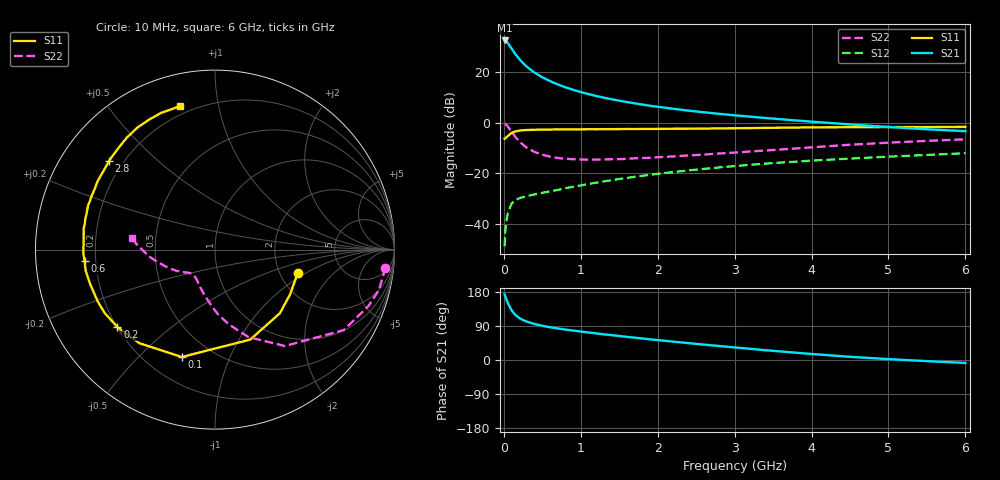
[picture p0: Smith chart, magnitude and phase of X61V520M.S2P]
! SIEMENS Small Signal Semiconductors
! BFP193W
! Si NPN RF Bipolar Junction Transistor in SOT343
! VCE = 1.5 V  IC = 20 mA
! Common Emitter S-Parameters:  April 1994
# GHz  S  MA  R  50
!  f  S11  S21  S12  S22
! GHz  MAG  ANG  MAG  ANG  MAG  ANG  MAG  ANG
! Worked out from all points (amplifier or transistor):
!   40 points, 10 MHz to 6 GHz, reference 50 ohm
!   highest |S21| = 32.5 dB at 10 MHz (marker M1)
!   |S21| within 3 dB of that: start of sweep to 96.08 MHz
!   unconditionally stable (mu >= 1): 873.5 MHz to 4.167 GHz
!   at 200 MHz: K = 0.36, MSG = 27.6 dB, |S12| = -30.0 dB
!   at 1.5 GHz: K = 1.13, MAG = 13.3 dB, |S12| = -22.3 dB
!   at 6 GHz: K = 0.95, MSG = 4.4 dB, |S12| = -12.1 dB
!   S11 on the Smith chart (normalised r, x): 10 MHz: 2.52, -0.84; 100 MHz: 0.34, -0.68; 200 MHz: 0.20, -0.34; 600 MHz: 0.16, -0.04; 2.8 GHz: 0.15, +0.36; 6 GHz: 0.16, +0.78
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0.01  0.4794 -15.5  42.23 173.0  0.0036 83.6  0.9545 -6.0
0.02  0.4869 -30.7  41.82 167.6  0.0073 77.8  0.9412 -13.7
0.03  0.5064 -44.4  40.79 161.7  0.0105 75.2  0.9115 -20.1
0.05  0.5384 -68.6  37.76 150.9  0.016 64.5  0.8462 -32.0
0.1  0.6264 -107.2  29.31 131.2  0.0249 50.1  0.6631 -54.1
0.15  0.671 -129.1  22.71 118.7  0.0294 42.0  0.5215 -69.1
0.2  0.6942 -141.6  18.13 110.8  0.0318 38.7  0.4261 -79.2
0.25  0.7091 -150.1  15.05 105.3  0.0338 37.4  0.3644 -86.9
0.3  0.7145 -156.2  12.72 101.2  0.0353 36.8  0.317 -93.1
0.4  0.722 -164.9  9.753 94.9  0.038 37.8  0.2627 -102.5
0.5  0.7298 -170.5  7.897 90.3  0.0408 40.1  0.2317 -109.6
0.6  0.7298 -175.0  6.608 86.5  0.0438 42.1  0.212 -115.3
0.8  0.7328 178.4  5 80.3  0.0504 46.4  0.1927 -123.0
1.1  0.7411 170.9  3.676 72.6  0.0612 50.2  0.185 -130.5
1.3  0.7427 166.5  3.118 67.7  0.0688 51.9  0.187 -133.6
1.6  0.7489 160.5  2.557 61.0  0.0806 53.3  0.1924 -137.2
2.2  0.757 150.0  1.882 48.5  0.1051 53.1  0.2145 -144.3
2.8  0.7695 140.1  1.491 36.9  0.1301 50.8  0.2452 -151.0
3.2  0.7801 133.9  1.314 29.6  0.1463 48.7  0.2684 -156.3
4.5  0.8125 116.5  0.922 8.4  0.1946 40.5  0.3653 -173.5
5.5  0.8184 107.7  0.739 -3.0  0.2298 34.2  0.4357 176.3
6  0.8233 103.6  0.678 -7.8  0.2482 31.3  0.4679 172.3
